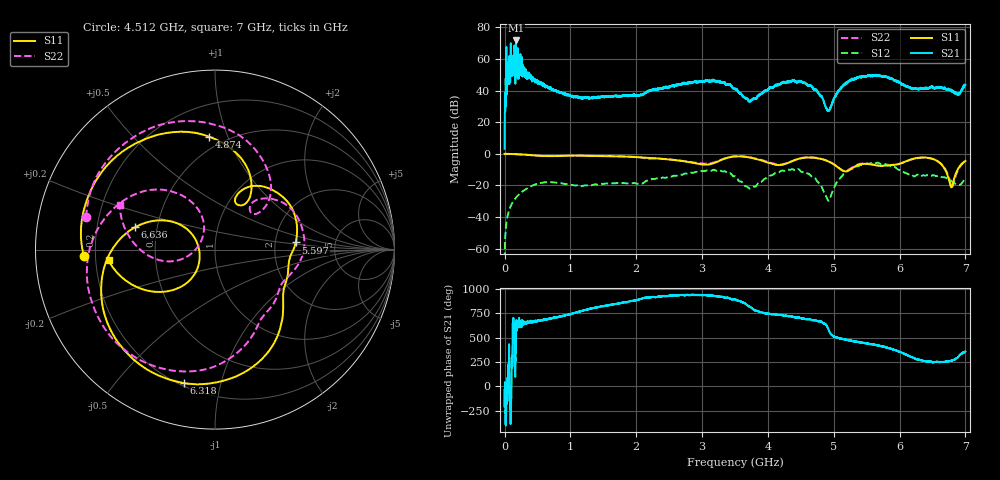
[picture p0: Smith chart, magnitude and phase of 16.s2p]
!Keysight Technologies,N5232A,MY52221221,A.10.65.11
!Date: Wednesday, October 16, 2024 12:06:01
!Correction: S11(Full 2 Port(1,4))
!S41(Full 2 Port(1,4))
!S14(Full 2 Port(1,4))
!S44(Full 2 Port(1,4))
!S2P File: Measurements: S11, S41, S14, S44:
# Hz S  RI  R 50
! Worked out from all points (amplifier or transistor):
!   4001 points, 300 kHz to 7 GHz, reference 50 ohm
!   highest |S21| = 71.6 dB at 173.5 MHz (marker M1)
!   |S21| within 3 dB of that: 94.58192 MHz to 94.92327 MHz (341.3 kHz wide, 0.36 % of centre)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
!   unconditionally stable (mu >= 1): nowhere
!   at 1.166 GHz: K = 3.13, MSG = 27.7 dB, |S12| = -20.4 dB
!   at 3.5 GHz: K = 11.06, MSG = 27.4 dB, |S12| = -14.1 dB
!   at 7 GHz: K = 12.72, MSG = 29.6 dB, |S12| = -15.5 dB
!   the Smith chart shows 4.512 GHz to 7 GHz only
!   S11 on the Smith chart (normalised r, x): 4.512 GHz: 0.16, -0.02; 4.874 GHz: 0.41, +0.86; 5.597 GHz: 2.62, +0.26; 6.318 GHz: 0.22, -0.77; 6.636 GHz: 0.37, +0.12; 7 GHz: 0.25, -0.05
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300000  -0.9966 -0.00934  1.153 -0.8526  -5.61e-05 8.45e-05  -0.9912 -0.0141
6.32973e7  -0.9716 0.2066  -733 307.8  0.00461 0.0144  -0.9683 0.2169
1.122952e8  -0.9216 0.3584  -274 -632.2  0.014 0.0229  -0.9124 0.3743
1.385441e8  -0.8838 0.43  -397 -565.9  0.0206 0.0258  -0.871 0.4515
1.735426e8  -0.8247 0.5232  -1746 3400  0.0309 0.0276  -0.8075 0.5482
2.10291e8  -0.7509 0.61  -92.62 -1148  0.0428 0.0262  -0.7266 0.6373
2.312901e8  -0.7053 0.6557  195.6 -452.3  0.0498 0.024  -0.6768 0.6838
3.27536e8  -0.4668 0.8108  98.09 -257.1  0.0781 -0.00246  -0.4199 0.8352
4.990286e8  -0.0222 0.8746  111.2 -131.8  0.0665 -0.0921  0.0497 0.873
1.1675e9  0.8462 -0.213  33.92 45.51  -0.0752 0.0591  0.802 -0.3503
2.3347e9  -0.6432 0.307  -103 -36.44  0.0108 -0.1643  -0.5489 0.4396
3.04517e9  0.2655 0.3679  -163.9 -130.8  -0.0181 0.2841  0.3697 0.316
3.50015e9  0.7956 -0.2442  -106.9 12.34  0.0223 -0.1949  0.7259 -0.4183
4.511607e9  -0.7298 -0.0367  175.9 -69.59  -0.1969 0.1799  -0.7173 0.1817
4.66735e9  -0.615 0.4529  99.59 -90.27  0.0427 0.1795  -0.4575 0.6244
4.873841e9  -0.0316 0.6287  2.786 -31.48  0.0472 -0.02  0.1653 0.6151
5.222076e9  0.1112 0.2739  -75.48 172.1  0.0961 0.2843  0.1959 0.2438
5.59656e9  0.4497 0.0401  90.1 275.7  0.0294 -0.4971  0.4408 -0.1137
5.83455e9  0.4014 -0.1587  209.6 130.2  -0.4297 0.1338  0.3337 -0.2876
6.317529e9  -0.1742 -0.7435  -0.5215 -117.7  -0.098 -0.1685  -0.4694 -0.5841
6.636016e9  -0.4459 0.1243  -46 -115  -0.0595 0.1753  -0.3374 0.3345
7e9  -0.5933 -0.0604  152 -6.891  0.0653 0.1544  -0.5311 0.2483
